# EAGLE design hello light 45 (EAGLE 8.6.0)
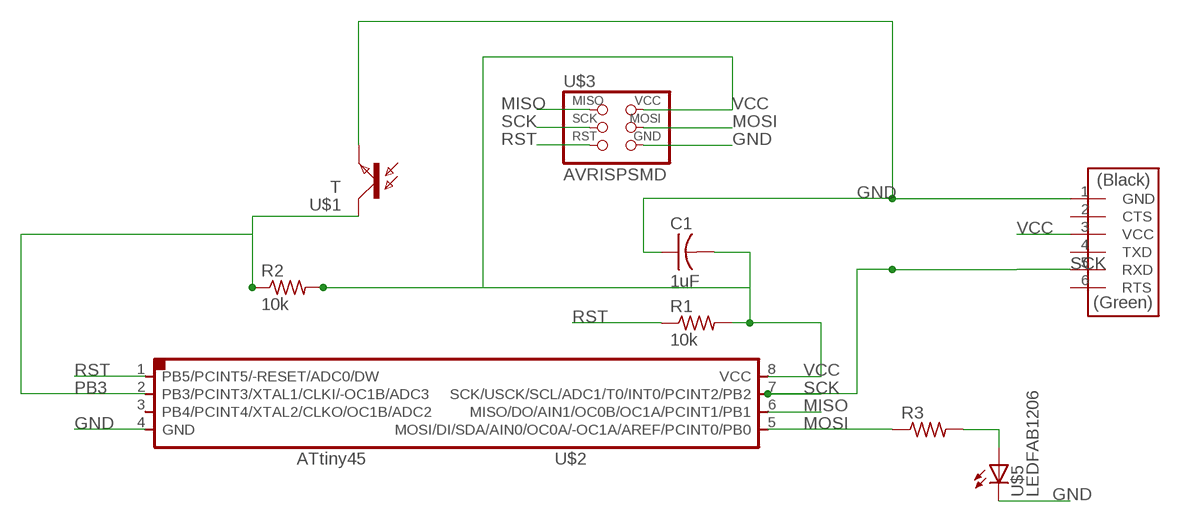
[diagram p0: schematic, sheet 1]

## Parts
C1  1uF  CAP-US1206FAB  [C1206FAB]
R1  10k  RES-US1206FAB  [R1206FAB]
R2  10k  RES-US1206FAB  [R1206FAB]
R3  RES-US1206FAB  [R1206FAB]
U$1  T  PHOTOTRANSISTOR-NPN1206  [OP1206]
U$2  ATTINY45SI  [SOIC8]
U$3  AVRISPSMD  [2X03SMD]
U$4  FTDI-SMD-HEADER  [1X06SMD]
U$5  LEDFAB1206  [LED1206FAB]

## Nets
GND: C1.1 U$1.EMITTER(E) U$2.4(GND) U$3.6(GND) U$4.1(GND) U$5.2(C)
MISO: U$2.6(MISO/DO/AIN1/OC0B/OC1A/PCINT1/PB1) U$3.1(MISO)
MOSI: R3.1 U$2.5(MOSI/DI/SDA/AIN0/OC0A/-OC1A/AREF/PCINT0/PB0) U$3.4(MOSI)
N$1: R3.2 U$5.1(A)
PB3: R2.1 U$1.COLLECTOR(C) U$2.2(PB3/PCINT3/XTAL1/CLKI/-OC1B/ADC3)
RST: R1.1 U$2.1(PB5/PCINT5/-RESET/ADC0/DW) U$3.5(RST)
SCK: U$2.7(SCK/USCK/SCL/ADC1/T0/INT0/PCINT2/PB2) U$3.3(SCK) U$4.5(RXD)
VCC: C1.2 R1.2 R2.2 U$2.8(VCC) U$3.2(VCC) U$4.3(VCC)
Unconnected: U$2.3(PB4/PCINT4/XTAL2/CLKO/OC1B/ADC2) U$4.2(CTS) U$4.4(TXD) U$4.6(RTS)

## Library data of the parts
C1 = fab:CAP-US
R1-R3 = fab:RES-US: Resistor (US Symbol)
U$1 = fab:PHOTOTRANSISTOR-NPN
U$2 = fab:ATTINY45
U$3 = fab:AVRISP
U$4 = fab:FTDI-SMD-HEADER
U$5 = fab:LED: LED

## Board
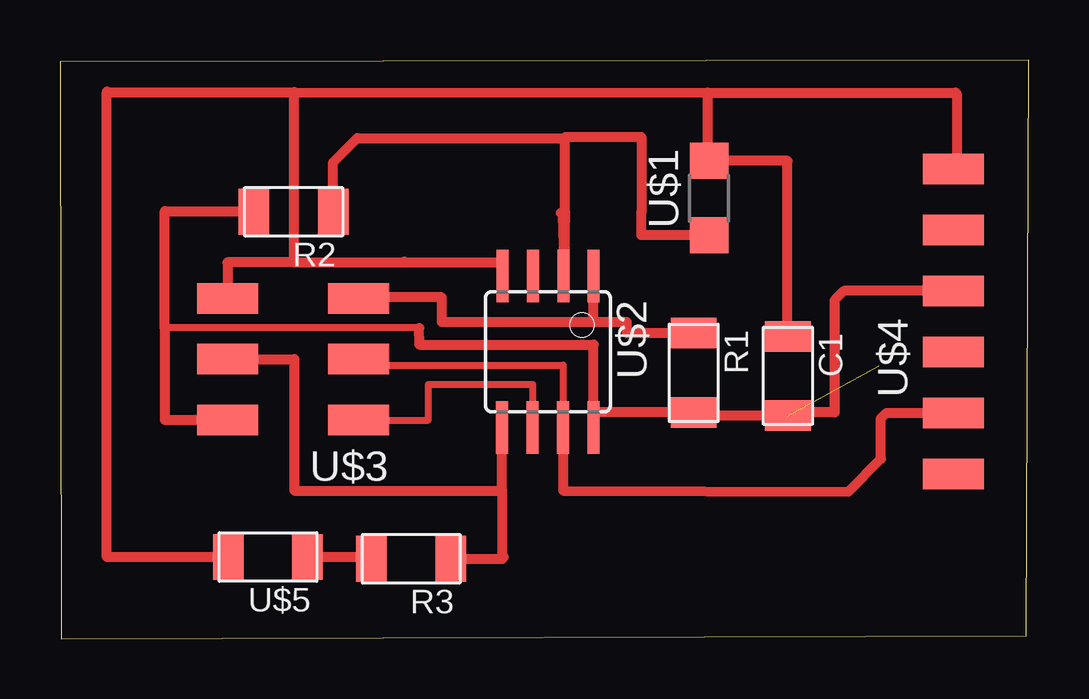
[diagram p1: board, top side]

Size 40.38 x 24.11 mm. Coordinates in mm from the lower left corner, seen from the top.
Outline: 0.06,0 40.28,0.13 40.38,24.11 0,24.04 0.06,0
Copper layers (1*16): Top 0.035mm / dielectric 1.5mm / Bottom 0.035mm
Design rules "default *": minimum track width 10mil, minimum drill 24mil, track to track 16mil, track to pad 16mil, pad to pad 16mil, via to via 16mil, smd to smd 16mil, copper to edge 40mil, drill to drill 8mil, minimum pad ring 10mil, minimum via ring 8mil, stop-mask expansion 4mil, vias tented up to drill 0mil, thermal gap 10mil

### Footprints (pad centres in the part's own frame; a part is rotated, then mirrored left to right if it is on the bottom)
C1206FAB = smd 1.27 x 1.905: 1 -1.651,0; 2 1.651,0
R1206FAB = smd 1.27 x 1.905: 1 -1.651,0; 2 1.651,0
OP1206 = smd 1.5 x 1.6: COLLECTOR -1.55,0; EMITTER 1.55,0
SOIC8 = smd 0.5 x 2.2: 1 -1.905,-3.154; 2 -0.645,-3.154; 3 0.625,-3.154; 4 1.895,-3.154; 5 1.905,3.154; 6 0.635,3.154; 7 -0.635,3.154; 8 -1.905,3.154
2X03SMD = smd 2.54 x 1.27: 1 -2.54,2.54; 2 2.92,2.54; 3 -2.54,0; 4 2.92,0; 5 -2.54,-2.54; 6 2.92,-2.54
1X06SMD = smd 2.54 x 1.27: 1 0,6.35; 2 0,3.81; 3 0,1.27; 4 0,-1.27; 5 0,-3.81; 6 0,-6.35
LED1206FAB = smd 1.27 x 1.905: 1 -1.651,0; 2 1.651,0

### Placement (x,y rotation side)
C1  30.34,10.95 270 top
R1  26.41,11.08 270 top
R2  9.74,17.79 180 top
R3  14.64,3.33 180 top
U$1  27.06,18.36 90 top
U$2  20.34,11.96 180 top
U$3  9.9,11.64 180 top
U$4  37.25,13.22 0 top
U$5  8.67,3.4 180 top

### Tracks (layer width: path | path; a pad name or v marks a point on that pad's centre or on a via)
GND
  Top 0.406: 9.76,15.68 6.98,15.68 U$3.6 | 9.76,15.68 14.38,15.68 | 14.38,15.68 18.45,15.68 U$2.4 | C1.1 30.33,12.6 30.33,19.91 U$1.EMITTER 27,19.97 27,22.76 | 36.91,19.91 U$4.1 37.6,19.57 37.77,19.74 37.38,20.13 37.38,22.71 37.34,22.75 27,22.76 | 9.76,22.77 9.77,22.77 27,22.76 | 9.76,15.68 9.76,22.77 | 14.35,15.71 14.38,15.68 | U$5.2 1.95,3.4 1.95,22.77 | 1.95,22.8 1.95,22.77 | 1.95,22.77 9.76,22.77
MISO
  Top 0.3: U$3.1 15.36,9.1 15.36,10.6 19.71,10.6 U$2.6
  Top 0.406: U$2.6 19.7,8.74 | 12.44,9.08 U$3.1
MOSI
  Top 0.406: U$3.4 9.76,11.64 9.76,6.17 18.44,6.17 | 18.44,6.17 U$2.5 | 18.44,6.17 18.44,3.4 | 18.44,3.4 18.5,3.4 | R3.1 18.44,3.33 18.44,3.4
N$1
  Top 0.406: R3.2 12.99,3.4 U$5.1
PB3
  Top 0.406: 21.04,17.79 20.98,17.65 | 20.98,17.65 21.06,17.79 20.87,17.75 | 21.04,17.79 U$2.2 21.04,15.11 | U$1.COLLECTOR 24.23,16.81 24.23,17.75 24.23,20.91 21.08,20.91 21.04,20.88 | 21.04,15.11 21.05,15.11 20.98,17.65 | 21.04,15.11 21.04,17.79 | 21.04,17.79 21.04,20.88 | R2.1 11.39,19.86 12.39,20.86 21.03,20.86 21.04,20.88
RST
  Top 0.406: R1.1 23.63,12.73 23.63,13.19 22.26,13.19 | 22.26,13.19 15.92,13.19 15.92,14.22 12.44,14.22 U$3.5 | 22.26,13.19 22.25,13.19 U$2.1
SCK
  Top 0.3: U$3.3 13.47,11.64 13.47,11.4 20.98,11.4 U$2.7
  Top 0.406: U$2.7 20.98,6.17 32.87,6.13 34.23,7.49 34.23,9.19 34.45,9.41 U$4.5 | 12.44,11.39 U$3.3
VCC  (1 unrouted)
  Top 0.3: 14.97,12.95 4.29,12.95 4.37,12.93
  Top 0.406: U$3.2 4.37,9.1 4.37,12.93 4.37,17.82 8.09,17.82 R2.2 | 14.97,12.95 14.98,12.25 22.25,12.25 22.25,9.43 | 22.25,9.43 U$2.8 | 22.25,9.43 R1.2 26.41,9.3 C1.2 30.48,9.43 32.29,9.43 32.29,14.1 32.68,14.49 U$4.3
